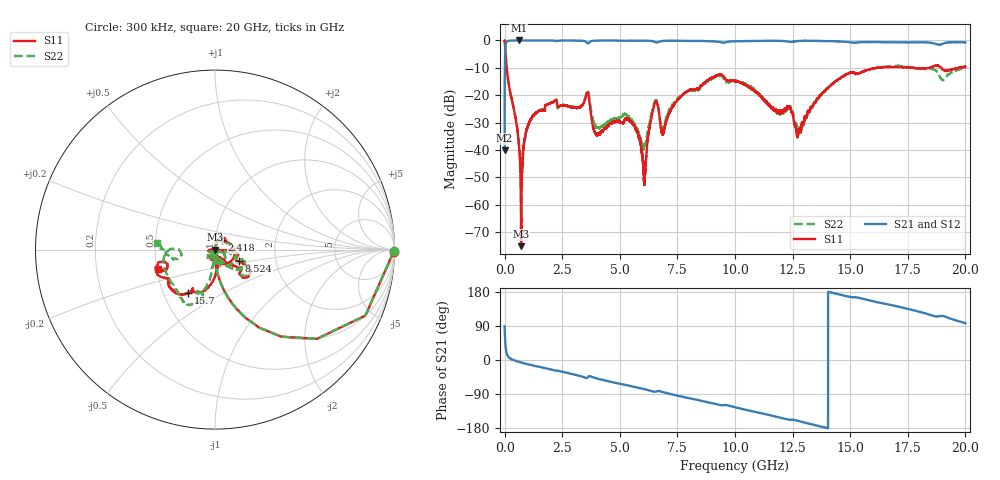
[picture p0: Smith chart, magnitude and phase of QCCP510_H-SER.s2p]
!{QCCP510}
!Johanson Technology Inc.
!www.johansontechnology.com
!Test Board Conditions:
!Substrate Type  RO4350B
!Substrate Thickness  20 mil
!Substrate Dk  3.66
!TL Type: GCPW
!TL Trace Width  36 mil
!TL Gap  12 mil
!Electrode orientation  Horizontal
!DUT TOPOLOGY	SERIES
!Mounting Pad LxW  26x36 mil
! Created Sat Jan  9 18:38:35 2021
# hz S ma R 50
! 2 Port Network Data from SP1.SP block
! freq  magS11  angS11  magS21  angS21  magS12  angS12  magS22  angS22
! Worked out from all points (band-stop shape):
!   20001 points, 300 kHz to 20 GHz, reference 50 ohm
!   highest |S21| = 0.00 dB at 617.3 MHz (marker M1); lowest = -40.1 dB at 300 kHz (marker M2)
!   |S21| within 3 dB of the highest: 30.55 MHz to end of sweep
!   lowest |S11| = -75.2 dB at 716.3 MHz (marker M3), VSWR 1.00, Z = 50 - j0.00401 ohm
!   |S11| at or under -10 dB: 89.7 MHz to 16.22 GHz (16.13 GHz wide, 198 % of centre); 17.73 GHz to 18.43 GHz (692.3 MHz wide, 3.83 % of centre); 18.96 GHz to 19.68 GHz (725.7 MHz wide, 3.76 % of centre)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
!   |S22| runs from -66.6 to 0.0 dB; largest |S21 - S12| = 0.018
!   S11 on the Smith chart (normalised r, x): 300 kHz: open; 2.418 GHz: 1.07, +0.11; 8.524 GHz: 1.30, -0.17; 15.7 GHz: 0.67, -0.35; 20 GHz: 0.51, -0.12
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300000  0.9955 -0.6  0.009862 88.6  0.009854 89.1  0.9957 -0.5
1.153e8  0.2492 -76.5  0.9673 13.3  0.9677 13.3  0.2499 -76.5
6.173e8  0.01317 -96.2  0.9999 -4.9  0.9986 -5.0  0.01346 -92.9
7.163e8  0.0001747 -166.7  0.9995 -6.6  0.9998 -6.6  0.0008446 -40.5
1.1683e9  0.03824 76.5  0.9986 -13.5  0.9983 -13.4  0.03751 74.5
2.4183e9  0.06448 53.1  0.9945 -29.9  0.9945 -29.9  0.06493 64.1
3.3343e9  0.06293 43.8  0.9888 -43.2  0.988 -43.2  0.06491 36.6
3.6063e9  0.1132 -23.7  0.886 -46.1  0.8855 -46.0  0.1244 -28.8
4.0293e9  0.01885 -157.6  0.9935 -49.2  0.9938 -49.2  0.0258 -97.2
5.4333e9  0.03345 -173.6  0.992 -68.2  0.9922 -68.3  0.03733 -136.1
6.0613e9  0.002313 105.8  0.9899 -76.9  0.9899 -76.9  0.01185 -72.6
6.4413e9  0.05319 -22.5  0.964 -82.9  0.9632 -83.0  0.05873 -28.1
6.6673e9  0.0591 -86.7  0.9354 -81.9  0.9356 -81.9  0.05929 -85.7
6.8793e9  0.01986 -37.1  0.9809 -84.8  0.9809 -84.9  0.02554 -37.2
8.5243e9  0.1494 -25.4  0.9782 -107.5  0.9767 -107.5  0.1433 -17.8
1.00003e10  0.1812 -36.5  0.9657 -124.7  0.9646 -124.7  0.1797 -35.7
1.23433e10  0.05952 -103.4  0.9462 -157.5  0.9495 -157.4  0.05748 -122.1
1.27503e10  0.02175 -106.4  0.9746 -160.9  0.9767 -160.8  0.02102 -139.0
1.33343e10  0.06098 -71.7  0.9829 -169.8  0.9852 -169.8  0.06172 -93.9
1.56973e10  0.2832 -122.1  0.9364 159.1  0.9396 158.9  0.2862 -104.0
1.66673e10  0.3241 -134.1  0.9234 146.5  0.9178 146.3  0.3366 -114.2
2e10  0.3326 -161.5  0.9212 97.2  0.9124 97.1  0.3256 173.0
